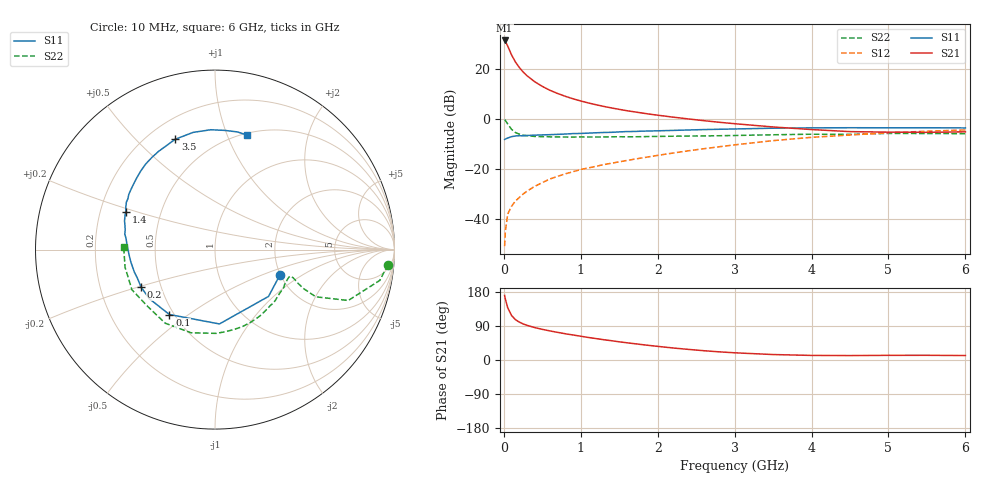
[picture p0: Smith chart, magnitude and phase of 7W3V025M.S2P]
! Infineon Technologies  Discrete & RF Semiconductors
! BFS17W
! Si NPN RF Bipolar Junction Transistor in SOT323
! VCE = 3 V  IC = 25 mA
! Common Emitter S-Parameters:  August  1999
# GHz  S  MA  R  50
!  f  S11  S21  S12  S22
! GHz  MAG  ANG  MAG  ANG  MAG  ANG  MAG  ANG
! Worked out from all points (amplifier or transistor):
!   36 points, 10 MHz to 6 GHz, reference 50 ohm
!   highest |S21| = 31.5 dB at 10 MHz (marker M1)
!   |S21| within 3 dB of that: start of sweep to 60.93 MHz
!   unconditionally stable (mu >= 1): 223.2 MHz to 2.333 GHz; 4.369 GHz to end of sweep
!   at 250 MHz: K = 1.05, MAG = 23.2 dB, |S12| = -30.1 dB
!   at 1.4 GHz: K = 1.20, MAG = 8.4 dB, |S12| = -17.8 dB
!   at 6 GHz: K = 1.08, MAG = -2.1 dB, |S12| = -4.4 dB
!   S11 on the Smith chart (normalised r, x): 10 MHz: 1.99, -0.66; 100 MHz: 0.47, -0.42; 200 MHz: 0.39, -0.21; 1.4 GHz: 0.31, +0.19; 3.5 GHz: 0.31, +0.66; 6 GHz: 0.52, +1.18
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0.01  0.3886 -21.2  37.74 170.4  0.0028 83.2  0.9674 -5.0
0.02  0.3962 -41.2  36.3 160.6  0.0056 82.3  0.934 -10.6
0.05  0.4149 -86.6  29.22 138.0  0.0123 66.8  0.7947 -20.9
0.1  0.442 -125.1  19.4 117.5  0.0177 59.4  0.6201 -25.1
0.15  0.4566 -143.1  14 106.6  0.0225 59.7  0.5358 -23.7
0.2  0.462 -153.1  10.86 100.1  0.0265 62.9  0.4973 -22.0
0.25  0.4607 -159.9  8.819 95.3  0.0311 63.8  0.4735 -20.5
0.3  0.4666 -164.5  7.413 91.6  0.0355 66.0  0.462 -19.8
0.4  0.4739 -171.6  5.618 85.6  0.0443 67.7  0.4471 -19.4
0.5  0.4795 -176.3  4.517 80.9  0.0529 69.4  0.4424 -19.8
0.6  0.4851 179.7  3.766 76.7  0.0626 70.3  0.4387 -20.9
0.7  0.4917 176.5  3.249 72.9  0.0708 70.7  0.4363 -22.6
0.9  0.5097 170.3  2.543 66.0  0.0875 71.8  0.4337 -26.6
1.1  0.5208 164.5  2.098 59.4  0.1043 71.7  0.4353 -31.4
1.4  0.5405 156.9  1.667 50.9  0.1295 71.9  0.4389 -39.5
1.8  0.5706 147.3  1.316 40.5  0.1657 72.2  0.4421 -51.6
2.2  0.5901 138.0  1.09 31.7  0.2075 71.4  0.4513 -63.8
2.8  0.6221 124.5  0.86 21.5  0.2773 67.8  0.4615 -83.2
3.5  0.6536 109.8  0.692 14.4  0.3677 61.0  0.4823 -106.1
4.5  0.6682 92.0  0.558 11.7  0.4771 47.6  0.4911 -140.1
5.5  0.6675 79.1  0.54 12.4  0.5681 34.8  0.5106 -168.9
6  0.6619 74.2  0.553 11.8  0.6035 28.7  0.509 178.4
